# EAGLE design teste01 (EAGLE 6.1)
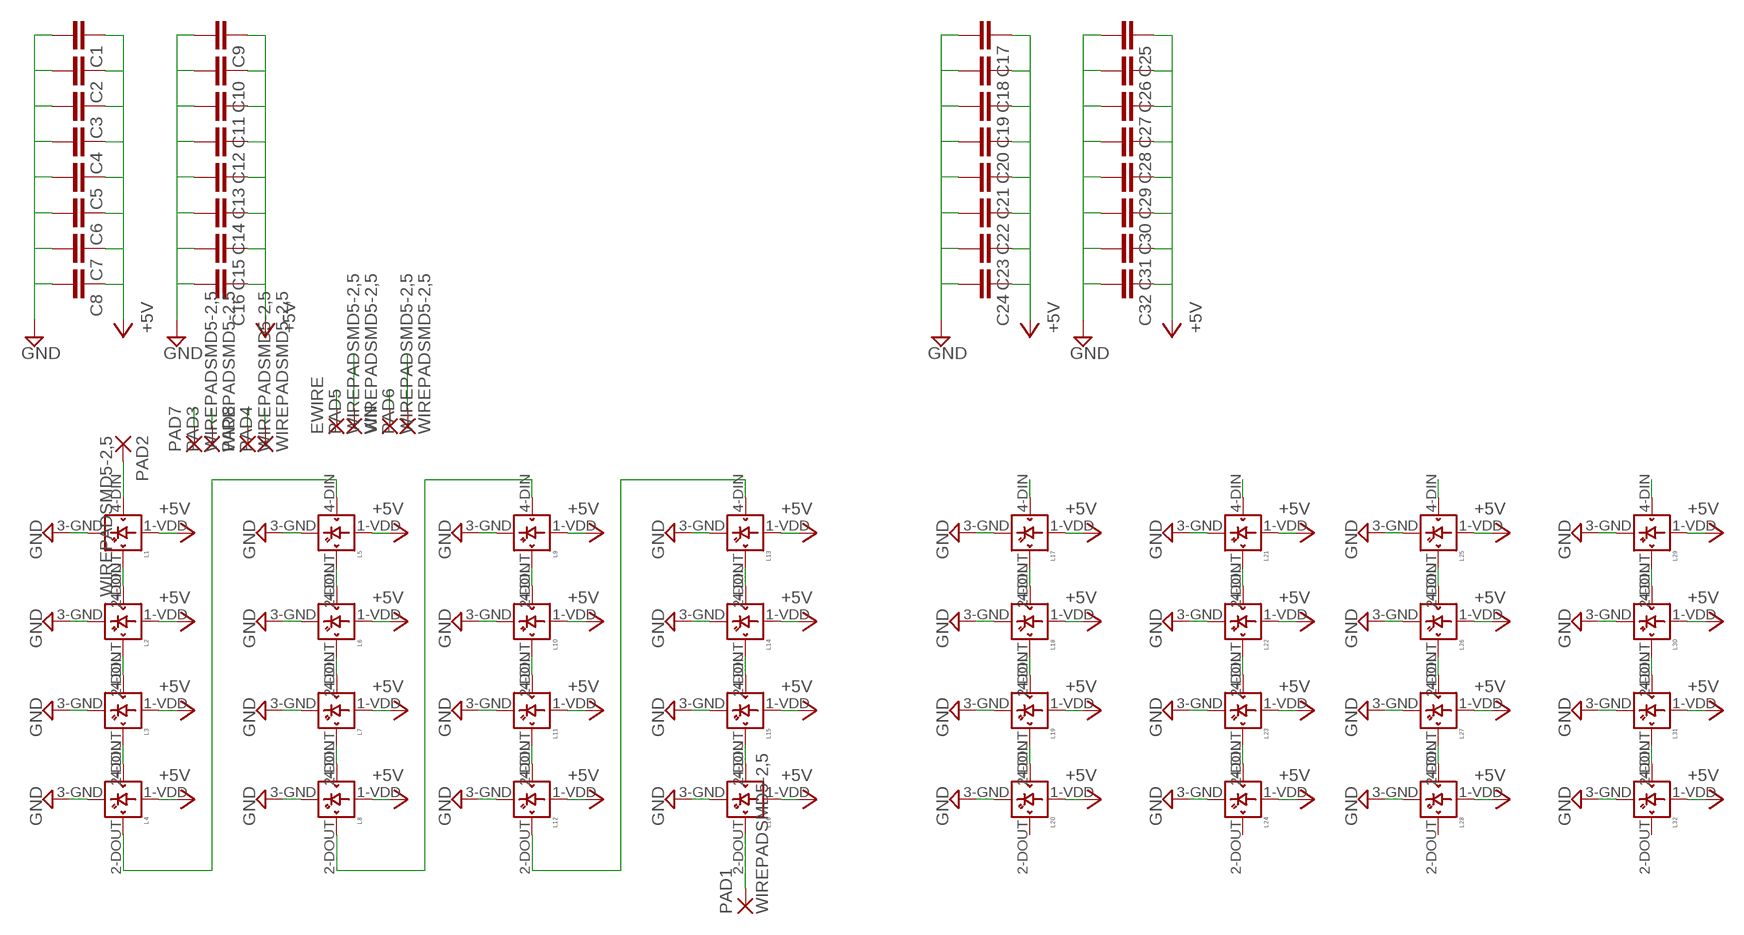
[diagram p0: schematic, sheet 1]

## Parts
C1  C-EUC0805K  [C0805K]
C2  C-EUC0805K  [C0805K]
C3  C-EUC0805K  [C0805K]
C4  C-EUC0805K  [C0805K]
C5  C-EUC0805K  [C0805K]
C6  C-EUC0805K  [C0805K]
C7  C-EUC0805K  [C0805K]
C8  C-EUC0805K  [C0805K]
C9  C-EUC0805K  [C0805K]
C10  C-EUC0805K  [C0805K]
C11  C-EUC0805K  [C0805K]
C12  C-EUC0805K  [C0805K]
C13  C-EUC0805K  [C0805K]
C14  C-EUC0805K  [C0805K]
C15  C-EUC0805K  [C0805K]
C16  C-EUC0805K  [C0805K]
C17  C-EUC0805K  [C0805K]
C18  C-EUC0805K  [C0805K]
C19  C-EUC0805K  [C0805K]
C20  C-EUC0805K  [C0805K]
C21  C-EUC0805K  [C0805K]
C22  C-EUC0805K  [C0805K]
C23  C-EUC0805K  [C0805K]
C24  C-EUC0805K  [C0805K]
C25  C-EUC0805K  [C0805K]
C26  C-EUC0805K  [C0805K]
C27  C-EUC0805K  [C0805K]
C28  C-EUC0805K  [C0805K]
C29  C-EUC0805K  [C0805K]
C30  C-EUC0805K  [C0805K]
C31  C-EUC0805K  [C0805K]
C32  C-EUC0805K  [C0805K]
EWIRE  WIREPADSMD5-2,5  [5-2,5]
L1  WS2812B  [WS2812B]
L2  WS2812B  [WS2812B]
L3  WS2812B  [WS2812B]
L4  WS2812B  [WS2812B]
L5  WS2812B  [WS2812B]
L6  WS2812B  [WS2812B]
L7  WS2812B  [WS2812B]
L8  WS2812B  [WS2812B]
L9  WS2812B  [WS2812B]
L10  WS2812B  [WS2812B]
L11  WS2812B  [WS2812B]
L12  WS2812B  [WS2812B]
L13  WS2812B  [WS2812B]
L14  WS2812B  [WS2812B]
L15  WS2812B  [WS2812B]
L16  WS2812B  [WS2812B]
L17  WS2812B  [WS2812B]
L18  WS2812B  [WS2812B]
L19  WS2812B  [WS2812B]
L20  WS2812B  [WS2812B]
L21  WS2812B  [WS2812B]
L22  WS2812B  [WS2812B]
L23  WS2812B  [WS2812B]
L24  WS2812B  [WS2812B]
L25  WS2812B  [WS2812B]
L26  WS2812B  [WS2812B]
L27  WS2812B  [WS2812B]
L28  WS2812B  [WS2812B]
L29  WS2812B  [WS2812B]
L30  WS2812B  [WS2812B]
L31  WS2812B  [WS2812B]
L32  WS2812B  [WS2812B]
PAD1  WIREPADSMD5-2,5  [5-2,5]
PAD2  WIREPADSMD5-2,5  [5-2,5]
PAD3  WIREPADSMD5-2,5  [5-2,5]
PAD4  WIREPADSMD5-2,5  [5-2,5]
PAD5  WIREPADSMD5-2,5  [5-2,5]
PAD6  WIREPADSMD5-2,5  [5-2,5]
PAD7  WIREPADSMD5-2,5  [5-2,5]
PAD8  WIREPADSMD5-2,5  [5-2,5]
VIN  WIREPADSMD5-2,5  [5-2,5]

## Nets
+5V: C1.1 C2.1 C3.1 C4.1 C5.1 C6.1 C7.1 C8.1 C9.1 C10.1 C11.1 C12.1 C13.1 C14.1 C15.1 C16.1 C17.1 C18.1 C19.1 C20.1 C21.1 C22.1 C23.1 C24.1 C25.1 C26.1 C27.1 C28.1 C29.1 C30.1 C31.1 C32.1 L1.1-VDD(VDD) L2.1-VDD(VDD) L3.1-VDD(VDD) L4.1-VDD(VDD) L5.1-VDD(VDD) L6.1-VDD(VDD) L7.1-VDD(VDD) L8.1-VDD(VDD) L9.1-VDD(VDD) L10.1-VDD(VDD) L11.1-VDD(VDD) L12.1-VDD(VDD) L13.1-VDD(VDD) L14.1-VDD(VDD) L15.1-VDD(VDD) L16.1-VDD(VDD) L17.1-VDD(VDD) L18.1-VDD(VDD) L19.1-VDD(VDD) L20.1-VDD(VDD) L21.1-VDD(VDD) L22.1-VDD(VDD) L23.1-VDD(VDD) L24.1-VDD(VDD) L25.1-VDD(VDD) L26.1-VDD(VDD) L27.1-VDD(VDD) L28.1-VDD(VDD) L29.1-VDD(VDD) L30.1-VDD(VDD) L31.1-VDD(VDD) L32.1-VDD(VDD)
GND: C1.2 C2.2 C3.2 C4.2 C5.2 C6.2 C7.2 C8.2 C9.2 C10.2 C11.2 C12.2 C13.2 C14.2 C15.2 C16.2 C17.2 C18.2 C19.2 C20.2 C21.2 C22.2 C23.2 C24.2 C25.2 C26.2 C27.2 C28.2 C29.2 C30.2 C31.2 C32.2 L1.3-GND(GND) L2.3-GND(GND) L3.3-GND(GND) L4.3-GND(GND) L5.3-GND(GND) L6.3-GND(GND) L7.3-GND(GND) L8.3-GND(GND) L9.3-GND(GND) L10.3-GND(GND) L11.3-GND(GND) L12.3-GND(GND) L13.3-GND(GND) L14.3-GND(GND) L15.3-GND(GND) L16.3-GND(GND) L17.3-GND(GND) L18.3-GND(GND) L19.3-GND(GND) L20.3-GND(GND) L21.3-GND(GND) L22.3-GND(GND) L23.3-GND(GND) L24.3-GND(GND) L25.3-GND(GND) L26.3-GND(GND) L27.3-GND(GND) L28.3-GND(GND) L29.3-GND(GND) L30.3-GND(GND) L31.3-GND(GND) L32.3-GND(GND) PAD3.1(P) PAD4.1(P) PAD7.1(P) PAD8.1(P)
N$1: L1.2-DOUT(DOUT) L2.4-DIN(DIN)
N$2: L2.2-DOUT(DOUT) L3.4-DIN(DIN)
N$3: L1.4-DIN(DIN) PAD2.1(P)
N$4: L3.2-DOUT(DOUT) L4.4-DIN(DIN)
N$5: L4.2-DOUT(DOUT) L5.4-DIN(DIN)
N$6: L5.2-DOUT(DOUT) L6.4-DIN(DIN)
N$7: L6.2-DOUT(DOUT) L7.4-DIN(DIN)
N$8: L7.2-DOUT(DOUT) L8.4-DIN(DIN)
N$9: L8.2-DOUT(DOUT) L9.4-DIN(DIN)
N$10: L9.2-DOUT(DOUT) L10.4-DIN(DIN)
N$11: L10.2-DOUT(DOUT) L11.4-DIN(DIN)
N$12: L11.2-DOUT(DOUT) L12.4-DIN(DIN)
N$13: L12.2-DOUT(DOUT) L13.4-DIN(DIN)
N$14: L13.2-DOUT(DOUT) L14.4-DIN(DIN)
N$15: L14.2-DOUT(DOUT) L15.4-DIN(DIN)
N$16: L15.2-DOUT(DOUT) L16.4-DIN(DIN)
N$17: L17.4-DIN(DIN)
N$18: L17.2-DOUT(DOUT) L18.4-DIN(DIN)
N$19: L18.2-DOUT(DOUT) L19.4-DIN(DIN)
N$20: L19.2-DOUT(DOUT) L20.4-DIN(DIN)
N$21: L21.4-DIN(DIN)
N$22: L21.2-DOUT(DOUT) L22.4-DIN(DIN)
N$23: L22.2-DOUT(DOUT) L23.4-DIN(DIN)
N$24: L23.2-DOUT(DOUT) L24.4-DIN(DIN)
N$25: L25.4-DIN(DIN)
N$26: L25.2-DOUT(DOUT) L26.4-DIN(DIN)
N$27: L26.2-DOUT(DOUT) L27.4-DIN(DIN)
N$28: L27.2-DOUT(DOUT) L28.4-DIN(DIN)
N$29: L29.4-DIN(DIN)
N$30: L29.2-DOUT(DOUT) L30.4-DIN(DIN)
N$31: L30.2-DOUT(DOUT) L31.4-DIN(DIN)
N$32: L31.2-DOUT(DOUT) L32.4-DIN(DIN)
N$33: L16.2-DOUT(DOUT) PAD1.1(P)
VIN: EWIRE.1(P) PAD5.1(P) PAD6.1(P) VIN.1(P)
Unconnected: L20.2-DOUT(DOUT) L24.2-DOUT(DOUT) L28.2-DOUT(DOUT) L32.2-DOUT(DOUT)

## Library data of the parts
C1-C32 = resistor:C-EU: CAPACITOR, European symbol
EWIRE PAD1-PAD8 VIN = wirepad:WIREPAD: Wire PAD connect wire on PCB
L1-L32 = adafruit:WS2812B

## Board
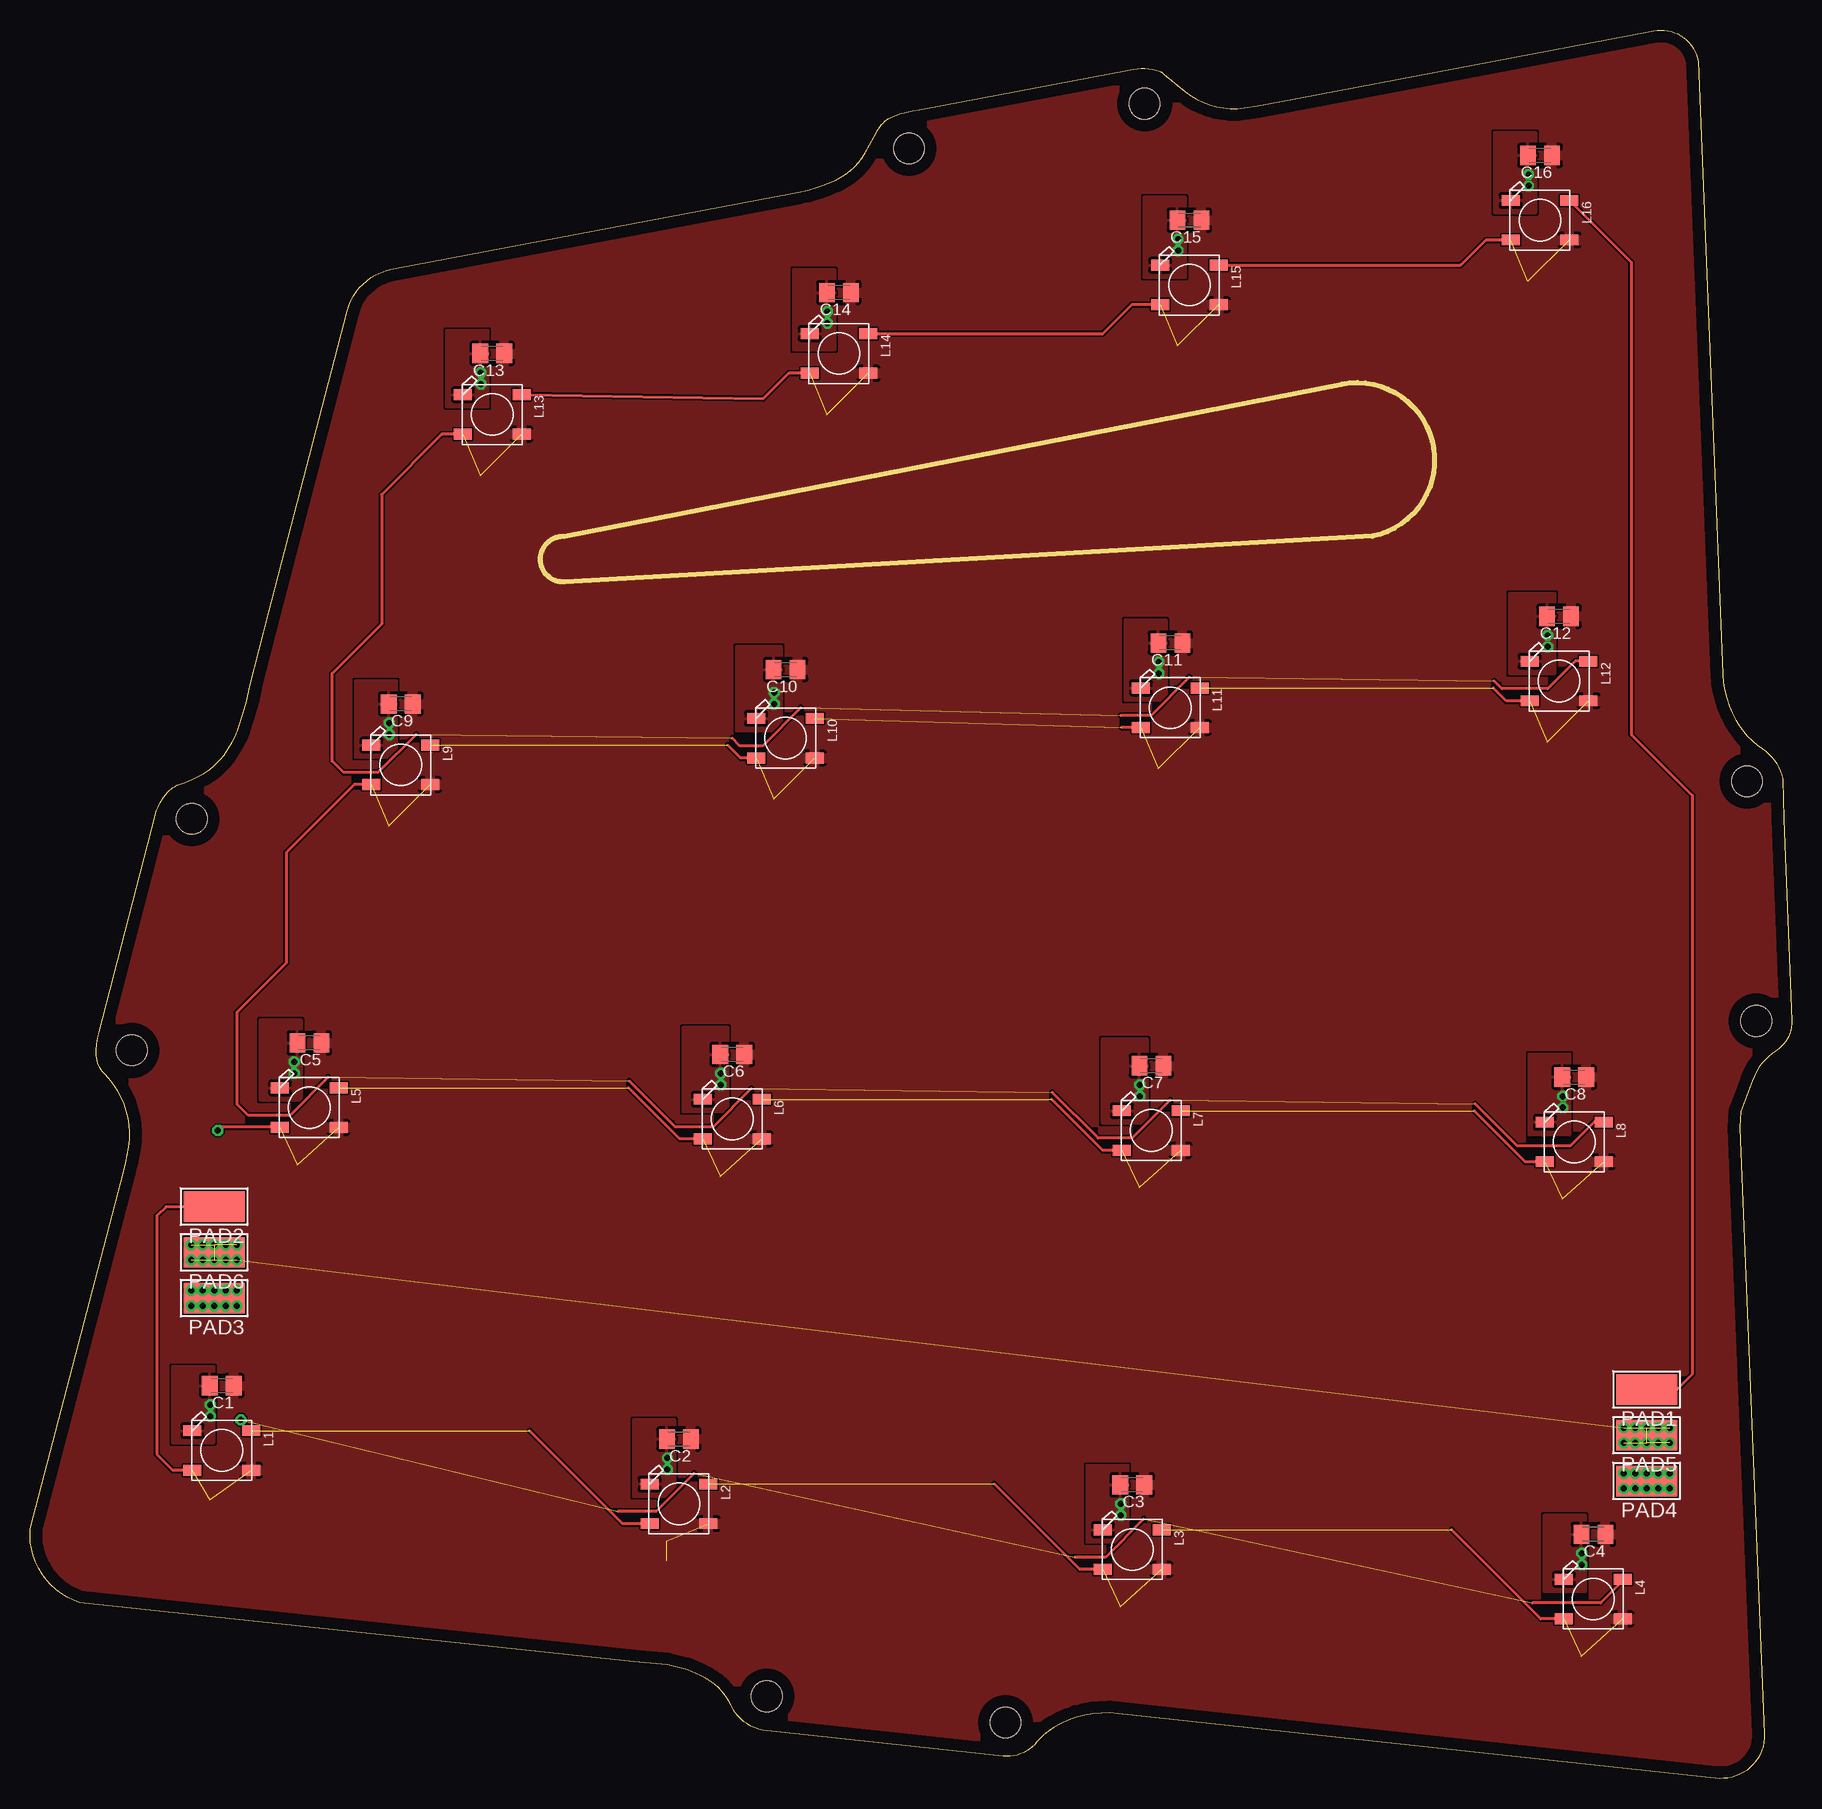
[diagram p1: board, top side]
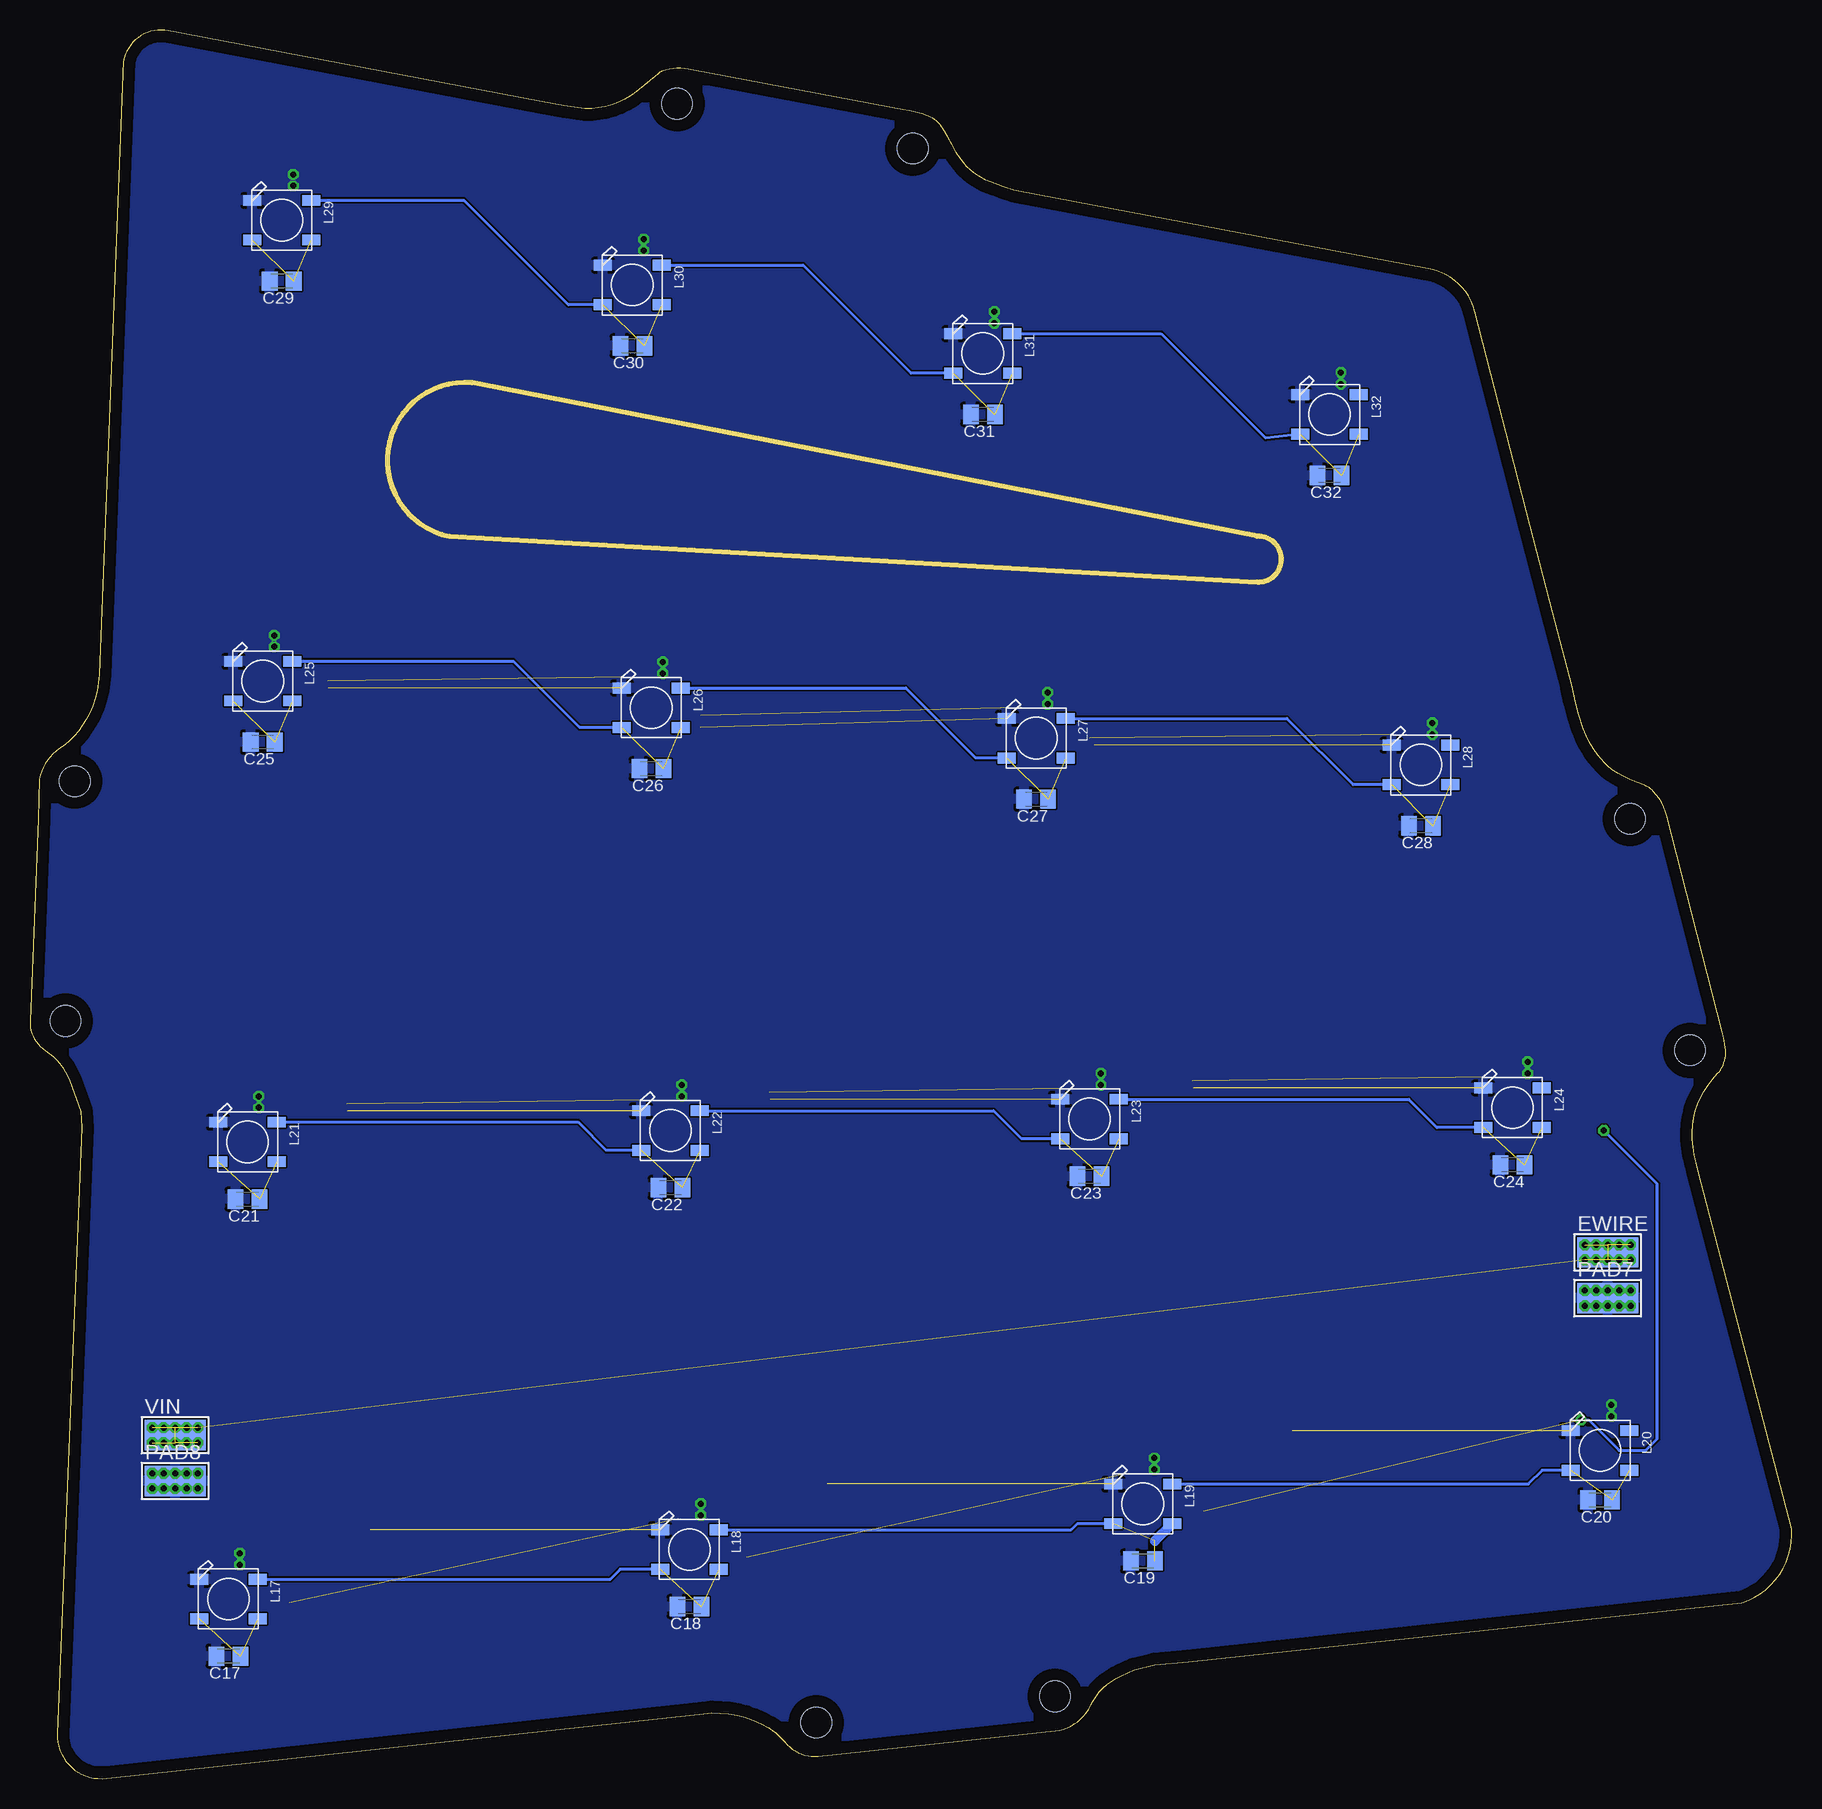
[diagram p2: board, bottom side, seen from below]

Size 146.81 x 145.75 mm. Coordinates in mm from the lower left corner, seen from the top.
Outline: 0.02,20.83 7.8,50.63 arc6 8.23,52.66 arc40 7.3,57.31 arc12 6.2,58.75 arc-48 5.52,60.7 arc-9 5.77,62.22 10.43,80.26 arc-28 11.53,82.29 arc-28 12.29,82.8 arc7 14.07,83.56 arc27 16.19,85.34 arc16 17.37,87.54 arc10 18.3,91.01 19.91,97.19 21.77,104.38 26.43,122.33 arc-64 30.07,125.8 64.02,132.24 arc14 67.15,133.25 arc35 69.6,135.54 arc0 70.71,137.49 arc-39 71.98,138.59 arc-16 74.09,139.09 91.95,142.48 arc-30 94.16,142.31 arc-35 94.49,142.06 96.27,140.62 arc47 101.18,139.26 arc4 104.57,139.86 135.3,145.7 arc-90 139.02,143.16 141.06,92.02 arc28 142.16,88.21 arc26 144.36,85.84 arc-44 146.05,83.3 146.14,80 146.81,63.16 arc-59 145.54,60.7 arc37 143.51,58.16 142.58,55.62 142.5,54.27 144.53,3.73 arc-95 140.8,0 90.68,5.42 arc37 85.27,4.23 arc21 83.91,3.05 arc-57 81.12,1.86 61.39,3.98 arc-59 58.43,6.1 arc42 55.89,8.55 54.79,9.06 53.1,9.48 50.3,9.74 4.16,14.65 arc-76 0.02,20.83
Copper layers (1*16): Top 0.035mm / dielectric 1.5mm / Bottom 0.035mm
Design rules: minimum track width 10mil, minimum drill 24mil, track to track 6mil, track to pad 6mil, pad to pad 6mil, via to via 6mil, smd to smd 6mil, copper to edge 40mil, drill to drill 8mil, minimum pad ring 10mil, minimum via ring 8mil, stop-mask expansion 4mil, vias tented up to drill 0mil, thermal gap 10mil
Holes 2.54 mm at 61.39,6.86 81.29,4.66 8.48,60.7 13.48,80 73.25,135.88 92.89,139.6 143.09,83.13 143.85,63.16
Milling: 4 lines

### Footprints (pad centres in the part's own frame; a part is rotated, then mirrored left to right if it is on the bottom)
C0805K = smd 1.3 x 1.6: 1 -1,0; 2 1,0
5-2,5 = smd 2.54 x 5.08: 1 0,0
WS2812B = smd 1.5 x 0.9: 1-VDD 2.45,-1.65; 2-DOUT 2.45,1.65; 3-GND -2.45,1.65; 4-DIN -2.45,-1.65

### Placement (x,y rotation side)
C1  15.98,32.74 180 top
C2  54.08,28.3 180 top
C3  91.86,24.49 180 top
C4  130.28,20.36 180 top
C5  23.28,61.32 180 top
C6  58.52,60.37 180 top
C7  93.45,59.41 180 top
C8  128.69,58.46 180 top
C9  30.9,89.58 180 top
C10  62.97,92.43 180 top
C11  95.03,94.66 180 top
C12  127.42,96.88 180 top
C13  38.52,118.79 180 top
C14  67.41,123.87 180 top
C15  96.62,129.9 180 top
C16  125.83,135.3 180 top
C17  130.28,10.2 180 bottom
C18  91.86,14.33 180 bottom
C19  54.08,18.14 180 bottom
C20  15.98,23.22 180 bottom
C21  128.69,48.3 180 bottom
C22  93.45,49.25 180 bottom
C23  58.52,50.21 180 bottom
C24  23.28,51.16 180 bottom
C25  127.42,86.4 180 bottom
C26  95.03,84.18 180 bottom
C27  62.97,81.64 180 bottom
C28  30.9,79.42 180 bottom
C29  125.83,124.82 180 bottom
C30  96.62,119.42 180 bottom
C31  67.41,113.71 180 bottom
C32  38.52,108.63 180 bottom
EWIRE  15.34,43.86 270 bottom
L1  15.98,27.35 0 top
L2  54.08,22.9 0 top
L3  91.86,19.09 0 top
L4  130.28,14.96 0 top
L5  23.28,55.92 0 top
L6  58.52,54.97 0 top
L7  93.45,54.02 0 top
L8  128.69,53.06 0 top
L9  30.9,84.5 0 top
L10  62.97,86.72 0 top
L11  95.03,89.26 0 top
L12  127.42,91.48 0 top
L13  38.52,113.71 0 top
L14  67.41,118.79 0 top
L15  96.62,124.5 0 top
L16  125.83,129.9 0 top
L17  130.28,14.96 0 bottom
L18  91.86,19.09 0 bottom
L19  54.08,22.9 0 bottom
L20  15.98,27.35 0 bottom
L21  128.69,53.06 0 bottom
L22  93.45,54.02 0 bottom
L23  58.52,54.97 0 bottom
L24  23.28,55.92 0 bottom
L25  127.42,91.48 0 bottom
L26  95.03,89.26 0 bottom
L27  62.97,86.72 0 bottom
L28  30.9,84.5 0 bottom
L29  125.83,129.9 0 bottom
L30  96.62,124.5 0 bottom
L31  67.41,118.79 0 bottom
L32  38.52,113.71 0 bottom
PAD1  134.72,32.43 90 top
PAD2  15.34,47.67 90 top
PAD3  15.34,40.05 90 top
PAD4  134.72,24.81 90 top
PAD5  134.72,28.62 90 top
PAD6  15.34,43.86 90 top
PAD7  15.34,40.05 270 bottom
PAD8  134.72,24.81 270 bottom
VIN  134.72,28.62 270 bottom

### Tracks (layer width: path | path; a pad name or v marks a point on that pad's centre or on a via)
+5V  (32 unrouted)
  Bottom 0.813: 53.08,19.8 L19.1-VDD
  pour Top (rank 2): -39.27,164.51 -39.27,-24.72 172.82,-24.72 172.82,164.51
GND  (via drill 0.5)  (2 unrouted)
  other vias: 37.57,116.25 37.57,117.2 66.46,121.33 66.46,122.28 95.67,128.31 95.67,127.36 124.88,133.71 124.88,132.76 15.02,31.16 15.02,30.2 53.12,26.71 53.12,25.76 90.91,22.9 90.91,21.95 129.32,18.77 129.32,17.82 127.74,56.87 127.74,55.92 92.49,57.83 92.49,56.87 57.57,58.78 57.57,57.83 22.01,59.73 22.01,58.78 126.47,95.29 126.47,94.34 94.08,93.07 94.08,92.12 62.01,90.53 62.01,89.58 29.95,87.99 29.95,87.04 17.25,40.68 16.29,40.68 15.34,40.68 14.39,40.68 13.44,40.68 13.44,39.41 14.39,39.41 15.34,39.41 16.29,39.41 17.25,39.41 136.63,24.17 135.67,24.17 134.72,24.17 133.77,24.17 132.82,24.17 136.63,25.44 135.67,25.44 134.72,25.44 133.77,25.44 132.82,25.44
  pour Bottom: -31.65,169.59 -31.65,-14.56 184.25,-14.56 184.25,169.59 -30.38,169.59
  pour Top: 34.71,120.69 34.71,114.34 38.2,114.34 38.2,120.69
  pour Top: 63.6,125.77 63.6,119.1 67.09,119.1 67.09,125.77
  pour Top: 92.81,131.8 92.81,125.14 96.3,125.14 96.3,131.8
  pour Top: 122.02,137.2 122.02,130.53 125.51,130.53 125.51,137.2
  pour Top: 123.29,98.78 123.29,92.12 127.1,92.12 127.1,98.78
  pour Top: 91.22,96.56 91.22,89.89 94.72,89.89 94.72,96.56
  pour Top: 58.84,94.34 58.84,87.35 62.65,87.35 62.65,94.34
  pour Top: 27.09,91.48 27.09,85.13 30.58,85.13 30.58,91.48
  pour Top: 19.15,63.22 19.15,56.56 22.64,56.56 22.64,63.22
  pour Top: 54.39,62.59 54.39,55.6 58.2,55.6 58.2,62.59
  pour Top: 89.32,61.64 89.32,54.65 93.13,54.65 93.13,61.64
  pour Top: 124.88,60.37 124.88,53.7 128.37,53.7 128.37,60.37
  pour Top: 126.15,21.95 126.15,15.6 129.64,15.6 129.64,21.95
  pour Top: 88.05,26.08 88.05,19.73 90.78,19.73 91.54,20.49 91.54,26.08
  pour Top: 11.85,34.33 11.85,27.98 15.34,27.98 15.34,34.33
  pour Top: 50.27,29.89 50.27,23.54 53,23.54 53.76,24.3 53.76,29.89
N$1  (1 unrouted)
  Top 0.254: 41.63,29 49.38,21.25 L2.4-DIN
N$2  (1 unrouted)
  Top 0.254: 80.37,24.55 87.48,17.44 L3.4-DIN
N$3
  Top 0.254: L1.4-DIN 11.91,25.7 10.58,27.03 10.58,46.91 11.34,47.67 PAD2.1
N$4  (1 unrouted)
  Top 0.254: 118.47,20.74 125.89,13.32 L4.4-DIN
N$5  (via drill 0.5)  (3 unrouted)
  Top 0.254: L4.2-DOUT 132.73,16.46 130.91,14.65 125.2,14.65 | 92.81,21.63 89.64,18.46 87.1,18.46 | 55.35,25.44 52.17,22.27 49,22.27 | v15.66,54.02 15.98,54.34 20.77,54.34 L5.4-DIN
  Bottom 0.254: v17.56,29.89 16.93,29.89 14.39,27.35 12.17,27.35 11.21,28.3 11.21,49.57 v15.66,54.02
N$6  (1 unrouted)
  Top 0.254: 49.89,57.57 54.14,53.32 L6.4-DIN
N$7  (1 unrouted)
  Top 0.254: 85.13,56.62 89.38,52.37 L7.4-DIN
N$8  (1 unrouted)
  Top 0.254: 120.37,55.67 124.62,51.42 L8.4-DIN
N$9  (3 unrouted)
  Top 0.254: L8.2-DOUT 130.34,54.71 128.37,52.75 123.93,52.75 120.43,56.24 | 95.03,56.56 91.86,53.38 89,53.38 85.19,57.19 | 60.11,57.51 56.93,54.34 53.76,54.34 49.95,58.14 | 24.87,58.46 21.69,55.29 18.2,55.29 17.25,56.24 17.25,63.86 21.37,67.99 21.37,77.19 27.03,82.85 L9.4-DIN
N$10  (1 unrouted)
  Top 0.254: L10.4-DIN 59.22,85.07 58.14,86.15
N$11  (1 unrouted)
  Top 0.254: L11.4-DIN 90.97,87.61
N$12  (1 unrouted)
  Top 0.254: L12.4-DIN 123.04,89.83 121.96,90.91
N$13  (3 unrouted)
  Top 0.254: L12.2-DOUT 128.75,93.13 126.47,90.85 122.66,90.85 122.02,91.48 | 96.62,91.8 93.45,88.63 90.91,88.63 | 64.24,89.26 61.06,86.08 59.16,86.08 58.52,86.72 | 32.17,87.04 28.99,83.86 26.14,83.86 25.18,84.81 25.18,92.12 29.31,96.25 29.31,107.04 34.33,112.06 L13.4-DIN
N$14
  Top 0.254: L13.2-DOUT 61.12,115.04 63.22,117.14 L14.4-DIN
N$15
  Top 0.254: L14.2-DOUT 89.38,120.44 91.8,122.85 L15.4-DIN
N$16
  Top 0.254: L15.2-DOUT 119.23,126.15 121.32,128.25 L16.4-DIN
N$18
  Bottom 0.254: L17.2-DOUT 98.46,16.61 97.64,17.44 L18.4-DIN
N$19
  Bottom 0.254: L18.2-DOUT 60.05,20.74 59.54,21.25 L19.4-DIN
N$20
  Bottom 0.254: L19.2-DOUT 21.95,24.55 20.8,25.7 L20.4-DIN
N$22
  Bottom 0.254: L21.2-DOUT 101.13,54.71 98.78,52.37 L22.4-DIN
N$23
  Bottom 0.254: L22.2-DOUT 66.52,55.67 64.17,53.32 L23.4-DIN
N$24
  Bottom 0.254: L23.2-DOUT 31.91,56.62 29.57,54.27 L24.4-DIN
N$26
  Bottom 0.254: L25.2-DOUT 106.53,93.13 101,87.61 L26.4-DIN
N$27
  Bottom 0.254: L26.2-DOUT 73.82,90.91 67.98,85.07 L27.4-DIN
N$28
  Bottom 0.254: L27.2-DOUT 42.07,88.37 36.55,82.85 L28.4-DIN
N$30
  Bottom 0.254: L29.2-DOUT 110.65,131.55 101.96,122.85 L30.4-DIN
N$31
  Bottom 0.254: L30.2-DOUT 82.4,126.15 73.38,117.14 L31.4-DIN
N$32
  Bottom 0.254: L31.2-DOUT 52.55,120.44 43.85,111.74 L32.4-DIN
N$33
  Top 0.254: L16.2-DOUT 133.45,126.38 133.45,87.04 138.53,81.96 138.53,33.7 137.26,32.43 PAD1.1
VIN  (via drill 0.5)  (23 unrouted)
  other vias: 17.25,44.49 16.29,44.49 15.34,44.49 14.39,44.49 13.44,44.49 13.44,43.22 14.39,43.22 15.34,43.22 16.29,43.22 17.25,43.22 136.63,29.25 135.67,29.25 134.72,29.25 133.77,29.25 132.82,29.25 132.82,27.98 133.77,27.98 134.72,27.98 135.67,27.98 136.63,27.98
